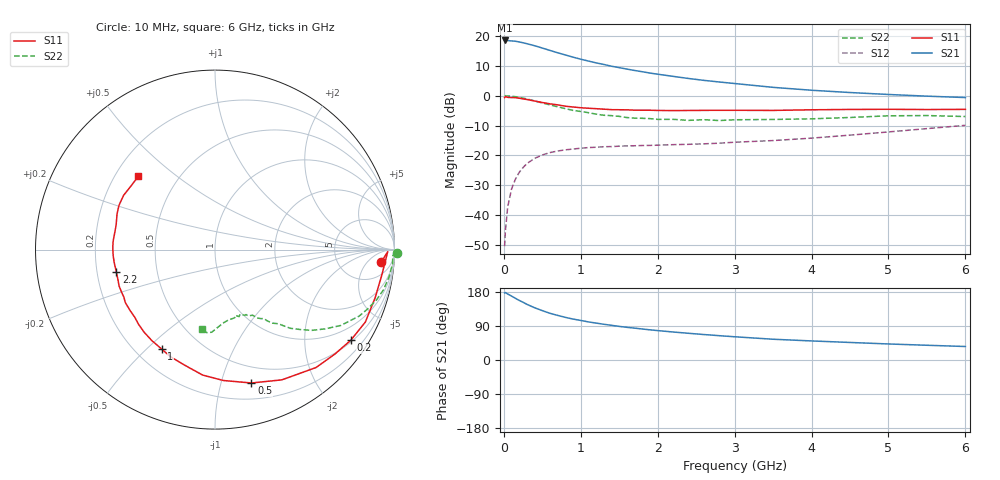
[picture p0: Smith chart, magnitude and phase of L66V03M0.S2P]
!  INFINEON TECHNOLOGIES Small Signal Semiconductors
! BFR380L3 , Si-NPN RF-Transistor in TSLP-3-1
!  Vce=6 V,  Ic=3 mA
! Common Emitter S-Parameters:  07. March 2005
#  GHz  S  MA  R  50
! f  S11  S21  S12  S22
! GHz  Mag  Ang  Mag  Ang  Mag  Ang  Mag  Ang
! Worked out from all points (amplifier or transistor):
!   36 points, 10 MHz to 6 GHz, reference 50 ohm
!   highest |S21| = 18.5 dB at 10 MHz (marker M1)
!   |S21| within 3 dB of that: start of sweep to 556.8 MHz
!   unconditionally stable (mu >= 1): 3.117 GHz to 4.463 GHz
!   at 250 MHz: K = 0.11, MSG = 20.9 dB, |S12| = -24.1 dB
!   at 1.4 GHz: K = 0.59, MSG = 13.5 dB, |S12| = -17.1 dB
!   at 6 GHz: K = 0.90, MSG = 4.7 dB, |S12| = -9.9 dB
!   S11 on the Smith chart (normalised r, x): 10 MHz: 14, -14; 200 MHz: 0.55, -3.22; 500 MHz: 0.34, -1.25; 1 GHz: 0.30, -0.56; 2.2 GHz: 0.28, -0.10; 6 GHz: 0.30, +0.37
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0.01  0.9298 -4.1  8.456 177.1  0.003 81.4  1.014 -1.0
0.02  0.9626 -0.7  8.4 178.0  0.0054 93.2  0.9911 -1.9
0.05  0.9401 -8.7  8.42 174.2  0.0136 87.4  0.9925 -4.5
0.1  0.9317 -16.8  8.301 168.7  0.0272 80.9  0.9813 -9.0
0.15  0.9299 -25.7  8.201 162.9  0.0397 75.8  0.9646 -13.5
0.2  0.9096 -33.7  7.984 157.2  0.0519 72.6  0.9425 -17.3
0.3  0.8652 -49.4  7.46 146.9  0.0729 64.6  0.8842 -24.8
0.4  0.8159 -62.8  6.901 137.9  0.089 57.7  0.8182 -31.1
0.5  0.7704 -74.7  6.31 130.3  0.1015 52.7  0.7566 -35.7
0.6  0.7309 -86.3  5.751 123.2  0.1115 48.2  0.7018 -39.9
0.7  0.7026 -95.6  5.254 117.7  0.1183 45.3  0.652 -43.1
0.9  0.647 -112.3  4.436 108.0  0.1277 40.5  0.5674 -48.2
1  0.629 -118.1  4.099 104.4  0.1317 39.3  0.5445 -49.4
1.1  0.6173 -124.7  3.815 100.5  0.1351 38.0  0.52 -52.0
1.3  0.5952 -135.8  3.347 94.3  0.1396 36.6  0.4705 -54.7
1.6  0.5804 -149.4  2.799 86.2  0.1443 35.9  0.4306 -59.5
2.2  0.5637 -167.4  2.114 73.9  0.1512 38.8  0.4021 -65.5
2.6  0.5684 -176.7  1.811 67.2  0.1561 42.1  0.3968 -70.2
3.5  0.5675 166.1  1.383 54.8  0.1771 49.9  0.4 -79.6
4.5  0.5891 155.2  1.132 46.3  0.2185 58.6  0.4318 -87.7
5.5  0.5871 143.2  0.984 38.9  0.2809 62.2  0.4651 -95.7
6  0.591 136.3  0.932 35.6  0.319 62.2  0.448 -99.6
